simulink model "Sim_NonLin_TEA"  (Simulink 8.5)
settings: Solver=ode45  StartTime=0.0  StopTime=100000  RelTol=1e-3
InitFcn:
  | start3
StopFcn:
  | Pl3
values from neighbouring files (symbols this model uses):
  ini = [wbo; atto; Hco]    [start.m]    (also in start1.m; start2.m; start3.m)
  Kpqr = lqr(sys,Q0,R0)    [des.m]
  nt = 12    [start.m]    (also in start1.m; start2.m; start3.m)
  r2d = 180/pi    (= 57.2957795131)    [start.m]    (also in start1.m; start2.m; start3.m)
  wo = 0.0011    [start.m]    (also in start1.m; start2.m; start3.m)
undefined symbols (not defined in the file or in its folder): Rigbod_Dynam_LVLH

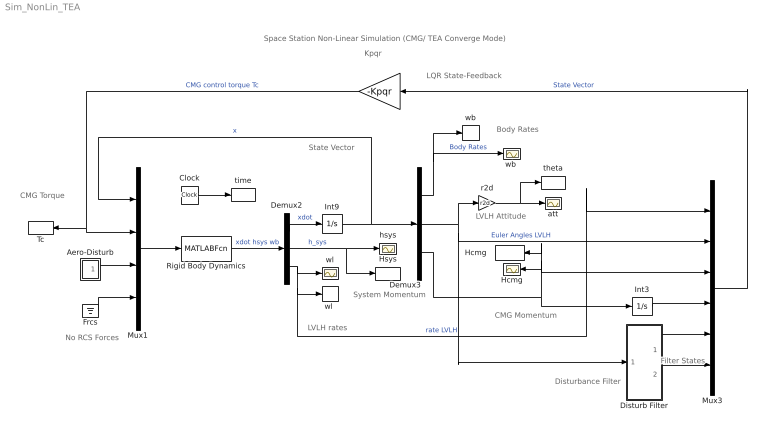
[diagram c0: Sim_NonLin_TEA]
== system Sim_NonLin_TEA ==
  note: Space Station Non-Linear Simulation (CMG/ TEA Converge Mode)
  note: LQR State-Feedback
  note: Kpqr
  note: CMG Torque
  note: LVLH rates
  note: System Momentum
  note: CMG Momentum
  note: Disturbance Filter
  note: Filter States
  note: Body Rates
  note: State Vector
  note: LVLH Attitude
  note: No RCS Forces
  " " : Gain  Gain=-Kpqr  Multiplication=Matrix(K*u)
  Aero-Disturb : Subsystem
  Clock : Clock
  Demux2 : Demux  Outputs=[9,3,3]
  Demux3 : Demux  Outputs=[3,3,3]
  Disturb Filter : Subsystem
  Frcs : Ground
  Hcmg : Scope
  "Hcmg  " : ToWorkspace  VariableName=Hcmg  SampleTime=-1
  Hsys : ToWorkspace  VariableName=Hsys  SampleTime=-1
  Int3 : Integrator
  Int9 : Integrator  InitialCondition=ini
  Mux1 : Mux  Inputs=[9, 3, 3, nt]
  Mux3 : Mux  Inputs=[3, 3, 3, 3, 1, 1]
  Rigid Body Dynamics : MATLABFcn  MATLABFcn=Rigbod_Dynam_LVLH( u(1:9), u(10:12), u(13:15), u(16:15+nt) )  OutputDimensions=15
  Tc : ToWorkspace  VariableName=Tcmg  SampleTime=-1
  att : Scope
  hsys : Scope
  r2d : Gain  Gain=r2d
  theta : ToWorkspace  VariableName=theta  SampleTime=-1
  time : ToWorkspace  VariableName=time  SampleTime=-1
  wb : ToWorkspace  VariableName=wb  SampleTime=-1
  "wb " : Scope
  wl : Scope
  "wl " : ToWorkspace  VariableName=wl  SampleTime=-1
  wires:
  Int3/1 -> Mux3/4
  Demux3/3 -> Int3/1, Hcmg/1, "Hcmg  "/1, Mux3/3
  Demux3/2 -> r2d/1, Mux3/2, Disturb Filter/1(the)  "Euler Angles LVLH"
  Demux2/2 -> hsys/1, Hsys/1  "h_sys"
  Mux1/1 -> Rigid Body Dynamics/1
  " "/1 -> Mux1/2, Tc/1  "CMG control torque Tc"
  Int9/1 -> Mux1/1, Demux3/1  "x"
  Demux2/1 -> Int9/1  "xdot"
  Rigid Body Dynamics/1 -> Demux2/1  "xdot hsys wb"
  Demux3/1 -> "wb "/1, wb/1  "Body Rates"
  Aero-Disturb/1(Td) -> Mux1/3
  r2d/1 -> att/1, theta/1
  Demux2/3 -> wl/1, "wl "/1, Mux3/1  "rate LVLH"
  Mux3/1 -> " "/1  "State Vector"
  Frcs/1 -> Mux1/4
  Clock/1 -> time/1
  Disturb Filter/1(a1) -> Mux3/5
  Disturb Filter/2(a2) -> Mux3/6

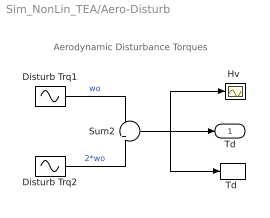
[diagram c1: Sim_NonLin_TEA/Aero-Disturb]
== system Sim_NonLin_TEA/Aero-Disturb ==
  note: Aerodynamic Disturbance Torques
  Disturb Trq1 : Sin  Amplitude=[1, 3, 1]  Bias="[1  8  1]"  Frequency=[wo, wo, wo]  SampleTime=0
  Disturb Trq2 : Sin  Amplitude=[1, 1, 1]*0.5  Frequency=[wo, wo, wo]*2  SampleTime=0
  "Hv " : Scope
  Sum2 : Sum  Inputs=+|+
  "Td " : ToWorkspace  VariableName=Td  SampleTime=-1
  Td : Outport
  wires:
  Disturb Trq2/1 -> Sum2/2  "2*wo"
  Sum2/1 -> Td/1, "Hv "/1, "Td "/1
  Disturb Trq1/1 -> Sum2/1  "wo"

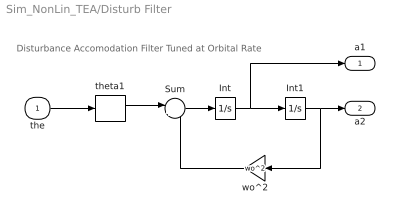
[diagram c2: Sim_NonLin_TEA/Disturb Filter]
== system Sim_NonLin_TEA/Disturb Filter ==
  note: Disturbance Accomodation Filter Tuned at Orbital Rate
  the : Inport
  Int : Integrator
  Int1 : Integrator
  Sum : Sum  Inputs=|+-
  theta1 : Selector  InputPortWidth=3  Indices=[2]
  wo^2 : Gain  Gain=wo^2
  a1 : Outport
  a2 : Outport  Port=2
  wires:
  Int/1 -> Int1/1, a1/1
  Sum/1 -> Int/1
  Int1/1 -> wo^2/1, a2/1
  wo^2/1 -> Sum/2
  theta1/1 -> Sum/1
  the/1 -> theta1/1
